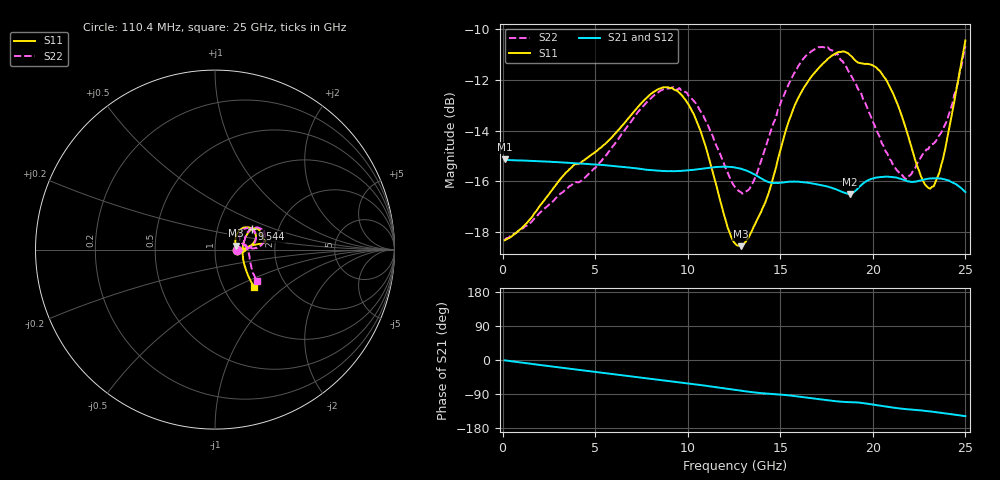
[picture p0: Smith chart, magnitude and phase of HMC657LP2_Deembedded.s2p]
! Hittite Microwave Corporation
! 2 Elizabeth Drive
! Chelmsford, MA 01824
! http://www.hittite.com
! Tel: 978-250-3343
! Fax: 978-250-3373
! Device:  HMC657LP2
! Description:  15 dB Wideband Fixed Attenuator
! Frequency:  DC - 25.00 GHz
! Package:  LP2  - 2x2 mm Dual Flatpack No-Lead (QFN) Plastic Package:  6 pin
! Ports:  2
!  Pin 1 = Ground
!  Pin 2 = RF1  = Port 1
!  Pin 3 = Ground
!  Pin 4 = Ground
!  Pin 5 = RF2  = Port 2
!  Pin 6 = Ground
! Data:  The device was measured on evaluation board 119194-1.
!  Data was collected using an calibrated network analyzer.
!  The evaluation circuit board was modeled and simulated.  This was use
!  to removed the evaluation board circuit from the measured data.
!  The reference plane is the center (edge) of the package pin.
! Misc:
! Date Measured:  2012-04-18
! Date:  2012-04-21 MJV
! Note:
!  Hittite supplies this data as a sample of measured data at the package pin for
!  for this package product.  Your particular data for this product may vary.
!  Data was taken at 25 degrees C.
!  Hittite reserves the right to change this data at anytime.
# GHz S DB R 50
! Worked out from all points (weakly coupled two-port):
!   249 points, 110.4 MHz to 25 GHz, reference 50 ohm
!   highest |S21| = -15.13 dB at 110.4 MHz (marker M1); lowest = -16.5 dB at 18.78 GHz (marker M2)
!   lowest |S11| = -18.5 dB at 12.86 GHz (marker M3), VSWR 1.27, Z = 63.1 + j2.8 ohm
!   |S11| at or under -10 dB: start of sweep to end of sweep
!   |S22| runs from -18.3 to -10.7 dB; largest |S21 - S12| = 0.00042
!   S11 on the Smith chart (normalised r, x): 110.4 MHz: 1.28, -0.00; 9.544 GHz: 1.47, +0.36; 25 GHz: 1.39, -0.63
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0.11036  -18.31 -0.7  -15.13 -0.9  -15.15 -0.9  -18.30 -0.4
4.32554  -15.20 -0.6  -15.30 -27.2  -15.30 -27.2  -15.91 -1.2
6.63386  -13.65 7.6  -15.44 -41.2  -15.44 -41.2  -13.95 4.4
8.44036  -12.36 19.0  -15.57 -52.0  -15.58 -52.0  -12.48 15.8
9.54434  -12.51 29.3  -15.59 -58.7  -15.59 -58.7  -12.33 25.1
10.64831  -13.93 37.4  -15.51 -65.7  -15.51 -65.7  -13.19 33.3
12.55518  -18.44 18.4  -15.45 -78.8  -15.45 -78.8  -16.22 28.1
12.85627  -18.55 10.7  -15.49 -80.9  -15.50 -80.9  -16.41 23.3
13.5588  -17.79 -2.3  -15.70 -85.3  -15.71 -85.3  -15.99 11.4
14.86349  -15.15 3.7  -16.06 -90.5  -16.06 -90.5  -13.19 1.6
15.76675  -13.03 6.9  -16.00 -95.1  -16.01 -95.1  -11.73 5.4
16.77036  -11.79 7.4  -16.09 -101.3  -16.09 -101.4  -10.84 13.6
18.07506  -10.93 8.9  -16.33 -109.1  -16.33 -109.1  -10.94 23.9
18.77759  -11.04 11.1  -16.49 -111.3  -16.49 -111.4  -11.78 28.4
19.98193  -11.43 24.1  -15.88 -117.5  -15.89 -117.5  -13.62 28.2
20.88518  -12.24 28.8  -15.82 -124.1  -15.82 -124.1  -15.10 19.7
21.78843  -13.93 26.1  -15.97 -129.7  -15.97 -129.7  -15.90 12.2
22.59133  -15.78 12.6  -15.96 -133.0  -15.96 -133.0  -15.06 6.0
23.09313  -16.28 -2.5  -15.88 -135.7  -15.89 -135.7  -14.59 -1.8
23.79566  -15.10 -24.3  -15.91 -140.1  -15.91 -140.1  -13.93 -15.8
24.29747  -13.25 -35.5  -16.04 -143.4  -16.02 -143.5  -12.94 -26.1
25  -10.45 -43.6  -16.42 -148.2  -16.41 -148.2  -10.68 -36.9
